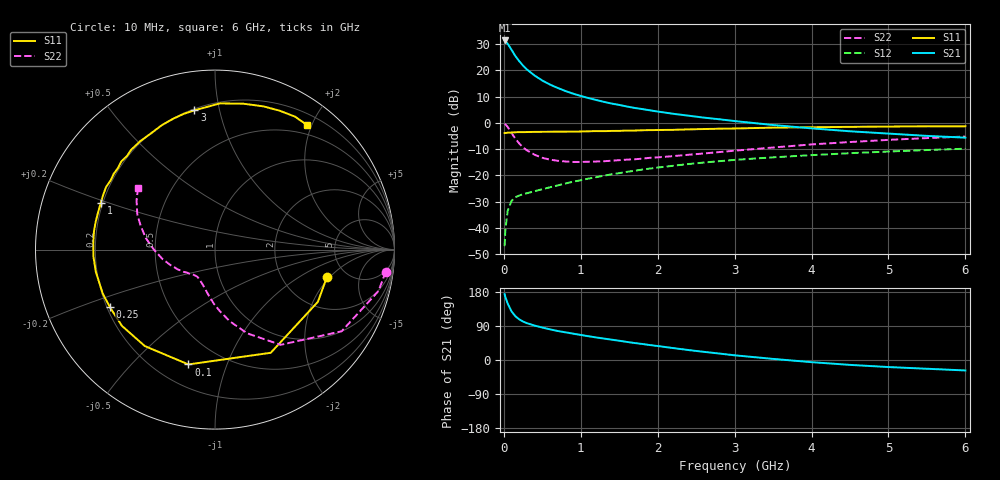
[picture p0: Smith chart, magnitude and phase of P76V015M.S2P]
! SIEMENS Small Signal Semiconductors
! BFP196
! Si NPN RF Bipolar Junction Transistor in SOT143
! VCE = 6 V  IC = 15 mA
! Common Emitter S-Parameters:  May  1996
# GHz  S  MA  R  50
!  f  S11  S21  S12  S22
! GHz  MAG  ANG  MAG  ANG  MAG  ANG  MAG  ANG
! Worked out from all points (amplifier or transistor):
!   36 points, 10 MHz to 6 GHz, reference 50 ohm
!   highest |S21| = 31.4 dB at 10 MHz (marker M1)
!   |S21| within 3 dB of that: start of sweep to 87.91 MHz
!   unconditionally stable (mu >= 1): 782.7 MHz to 3.384 GHz
!   at 250 MHz: K = 0.50, MSG = 24.5 dB, |S12| = -27.1 dB
!   at 1.4 GHz: K = 1.12, MAG = 11.4 dB, |S12| = -19.6 dB
!   at 6 GHz: K = 0.97, MSG = 2.1 dB, |S12| = -9.8 dB
!   S11 on the Smith chart (normalised r, x): 10 MHz: 3.55, -1.86; 100 MHz: 0.33, -0.74; 250 MHz: 0.21, -0.25; 1 GHz: 0.19, +0.19; 3 GHz: 0.21, +0.84; 6 GHz: 0.36, +1.94
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0.01  0.642 -13.9  37.26 173.7  0.0045 84.7  0.9593 -7.4
0.02  0.6429 -26.9  35.87 166.1  0.0094 77.0  0.9397 -14.2
0.05  0.6534 -61.6  32.24 148.9  0.0212 64.4  0.8397 -32.8
0.1  0.6567 -103.0  24.74 128.2  0.0328 48.6  0.6445 -55.4
0.15  0.6647 -126.0  18.77 115.5  0.0386 41.9  0.4996 -69.0
0.2  0.6705 -140.7  15.05 107.3  0.0414 38.5  0.4073 -78.4
0.25  0.6676 -151.2  12.32 101.4  0.0441 37.2  0.3422 -85.7
0.3  0.6717 -158.5  10.44 97.2  0.0458 38.0  0.3016 -91.2
0.4  0.6754 -169.3  7.996 90.8  0.0502 39.2  0.2479 -99.6
0.5  0.6784 -176.7  6.426 85.6  0.0547 41.3  0.2167 -106.3
0.6  0.6793 177.1  5.388 80.9  0.0596 43.8  0.2001 -111.7
0.7  0.6821 171.3  4.643 76.5  0.0646 44.8  0.1905 -116.0
0.8  0.6825 167.0  4.059 73.1  0.0702 46.2  0.1846 -119.7
1  0.6876 157.6  3.267 66.1  0.0812 47.8  0.1808 -125.3
1.1  0.6936 153.9  2.981 62.7  0.0871 48.4  0.1826 -128.0
1.6  0.7168 136.7  2.055 47.7  0.1171 47.6  0.2001 -139.4
2.2  0.7393 118.8  1.495 31.5  0.1529 43.2  0.2335 -151.4
3  0.7843 98.4  1.087 12.4  0.1978 34.8  0.2962 -169.5
3.5  0.8149 88.1  0.913 2.9  0.2215 29.0  0.3408 179.9
4.5  0.8425 71.3  0.694 -12.9  0.2657 18.0  0.4334 162.5
5.5  0.8646 59.0  0.567 -23.1  0.305 7.2  0.5152 148.0
6  0.863 53.4  0.525 -27.6  0.3232 1.3  0.5506 141.2
